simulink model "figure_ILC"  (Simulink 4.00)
settings: Solver=ode45  StartTime=0.0  StopTime=10.0  RelTol=1e-3
libraries: cstblocks x3

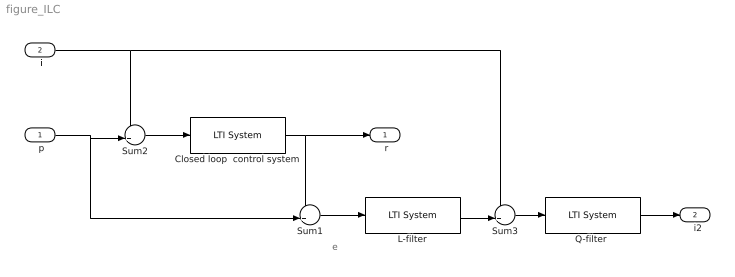
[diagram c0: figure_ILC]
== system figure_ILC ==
  note: e
  " p" : Inport  Port=1  LatchInput=off
  " i" : Inport  Port=2  LatchInput=off
  " L-filter " : cstblocks/LTI System  sys=L_d  IC=[]
  Closed loop  control system : cstblocks/LTI System  sys=Gcl  IC=[]
  "Q-filter " : cstblocks/LTI System  sys=Qd  IC=[]
  Sum1 : Sum  Inputs=-+|  SaturateOnIntegerOverflow=on
  Sum2 : Sum  Inputs=++|  SaturateOnIntegerOverflow=on
  Sum3 : Sum  Inputs=++|  SaturateOnIntegerOverflow=on
  " r" : Outport  Port=1
  "  i2" : Outport  Port=2
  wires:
  " i"/1 -> Sum2/1, Sum3/1
  " p"/1 -> Sum2/2, Sum1/2
  Sum2/1 -> Closed loop  control system/1
  Closed loop  control system/1 -> " r"/1, Sum1/1
  Sum1/1 -> " L-filter "/1
  " L-filter "/1 -> Sum3/2
  Sum3/1 -> "Q-filter "/1
  "Q-filter "/1 -> "  i2"/1
